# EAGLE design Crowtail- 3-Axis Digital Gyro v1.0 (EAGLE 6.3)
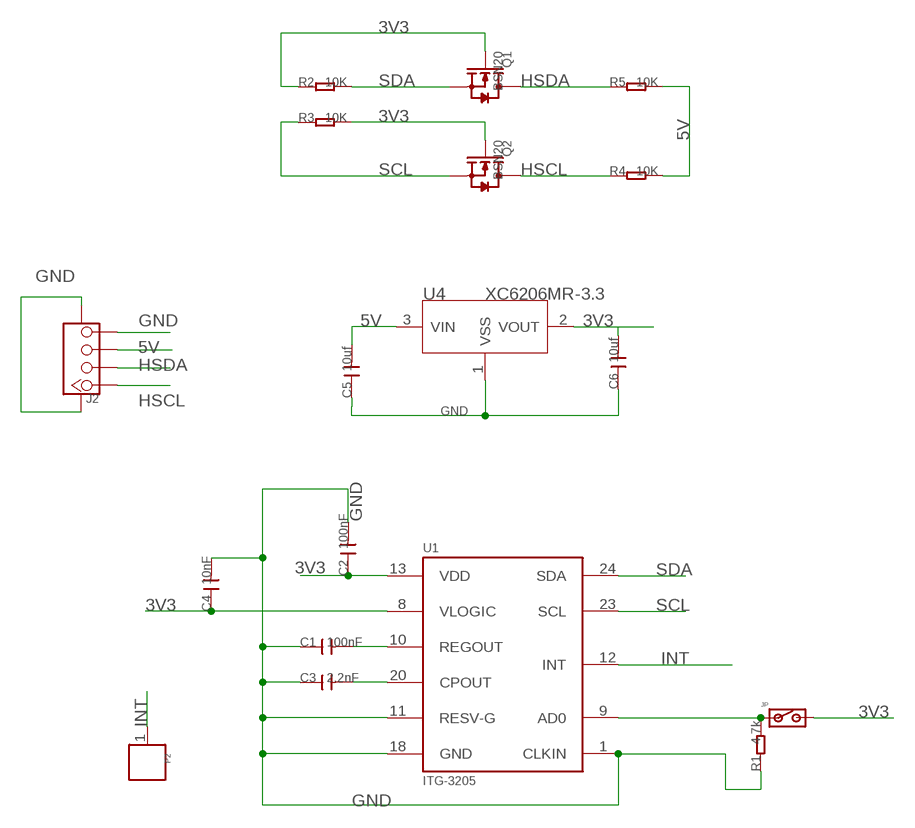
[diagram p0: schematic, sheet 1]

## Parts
C1  100nF  C-0603  [C0603]
C2  100nF  C-0603  [C0603]
C3  2.2nF  C-0603  [C0603]
C4  10nF  C-0603  [C0603]
C5  10uf  C-0603  [C0603]
C6  10uf  C-0603  [C0603]
J2  TWIG-4P-2.0-SMD-FEMALE-REINFORCE'DD'  [4P-SMD-2.0]
JP  DNP  JP_SW  [JP_SW]
P2  DNP  PAD'60/30'  [1P-65/35MIL]
Q1  BSN20  MOSFET-N'SOT23'  [SOT23]
Q2  BSN20  MOSFET-N'SOT23'  [SOT23]
R1  4.7k  R-0603  [R0603]
R2  10K  R-0603  [R0603]
R3  10K  R-0603  [R0603]
R4  10K  R-0603  [R0603]
R5  10K  R-0603  [R0603]
U1  ITG-3205  ITG-3200  [QFN-24]
U4  XC6206MR-3.3  XC6206MR  [SOT23]

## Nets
3V3: C2.1 C4.1 C6.2 JP.2 Q1.1(G) Q2.1(G) R2.1 R3.2 U1.8(VLOGIC) U1.13(VDD) U4.2(VOUT)
5V: C5.2 J2.3 R4.2 R5.2 U4.3(VIN)
GND: C1.1 C2.2 C3.1 C4.2 C5.1 C6.1 J2.4 J2.SS1 J2.SS2 R1.1 U1.1(CLKIN) U1.11(RESV-G) U1.18(GND) U4.1(VSS)
HSCL: J2.1 Q2.3(D) R4.1
HSDA: J2.2 Q1.3(D) R5.1
INT: P2.1 U1.12(INT)
N$2: C3.2 U1.20(CPOUT)
N$3: C1.2 U1.10(REGOUT)
N$4: JP.1 R1.2 U1.9(AD0)
SCL: Q2.2(S) R3.1 U1.23(SCL)
SDA: Q1.2(S) R2.2 U1.24(SDA)

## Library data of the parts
C1-C6 = Discrete:C*: Ceramic Capacitors
J2 = Connector:TWIG-4P-2.0-SMD-FEMALE-REINFORCE
JP = CPT_SMD:JP_SW
P2 = Discrete:PAD
Q1 Q2 = Discrete:MOSFET-N: IRLL014: http://www.vishay.com/docs/91319/sihll014.pdf
R1-R5 = Discrete:R*
U1 = IC:ITG-3200: ITG-3200 3-axis gyro, digital output, qfn24 package
U4 = IC:XC6206: LOW ESR Cap.Compatible Positive Voltage Regulators

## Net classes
0 default: width 0.203 mm, drill 0.305 mm, clearance 0.203 mm

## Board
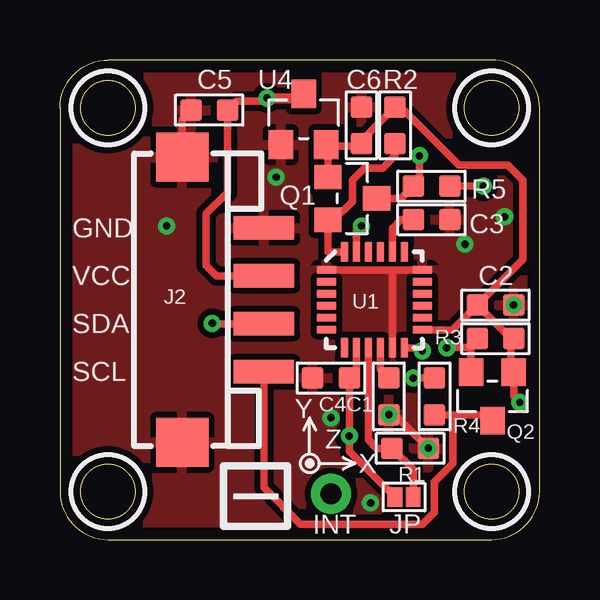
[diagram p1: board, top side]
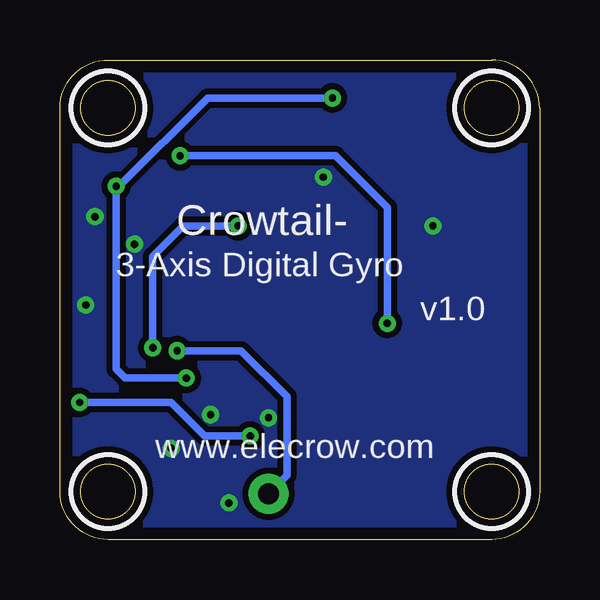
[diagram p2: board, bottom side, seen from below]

Size 20 x 20 mm. Coordinates in mm from the lower left corner, seen from the top.
Outline: 0,18 0,2 arc90 2,0 18,0 arc90 20,2 20,18 arc90 18,20 2,20 arc90 0,18
Outline: circle at 2,18 radius 1.14
Outline: circle at 2,2 radius 1.14
Outline: circle at 18,18 radius 1.14
Outline: circle at 18,2 radius 1.14
Copper layers (1*16): Top 0.035mm / dielectric 1.5mm / Bottom 0.035mm
Design rules "default *": minimum track width 10mil, minimum drill 12mil, track to track 8mil, track to pad 8mil, pad to pad 8mil, via to via 8mil, smd to smd 8mil, copper to edge 20mil, drill to drill 8mil, minimum pad ring 10mil, minimum via ring 8mil, stop-mask expansion 4mil, vias tented up to drill 100mil, thermal gap 10mil
tRestrict: area 0.5,16.5 to 3.5,19.5; area 0.5,0.5 to 3.5,3.5; area 16.5,16.5 to 19.5,19.5; area 16.5,0.5 to 19.5,3.5
bRestrict: area 0.5,16.5 to 3.5,19.5; area 0.5,0.5 to 3.5,3.5; area 16.5,16.5 to 19.5,19.5; area 16.5,0.5 to 19.5,3.5

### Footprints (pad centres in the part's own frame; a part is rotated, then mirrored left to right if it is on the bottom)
C0603 = smd 0.889 x 0.889: 1 -0.762,0; 2 0.762,0
4P-SMD-2.0 = smd 0.965 x 2.54: 1 -3,0; 2 -1,0; 3 1,0; 4 3,0 | smd 2.032 x 2.184: SS1 -5.946,3.4; SS2 5.946,3.4
JP_SW = smd 0.813 x 0.61: 1 0,0.381; 2 0,-0.381
1P-65/35MIL = drill 0.889 pad 1.651: 1 0,0
SOT23 = smd 1.016 x 1.143: 1 -0.889,-1.016; 2 0.889,-1.016; 3 0,1.016
R0603 = smd 0.889 x 0.889: 1 -0.762,0; 2 0.762,0
QFN-24 = smd 0.8 x 0.3: 1 -2,1.25; 2 -2,0.75; 3 -2,0.25; 4 -2,-0.25; 5 -2,-0.75; 6 -2,-1.25; 13 2,-1.25; 14 2,-0.75; 15 2,-0.25; 16 2,0.25; 17 2,0.75; 18 2,1.25 | smd 0.3 x 0.8: 7 -1.25,-2; 8 -0.75,-2; 9 -0.25,-2; 10 0.25,-2; 11 0.75,-2; 12 1.25,-2; 19 1.25,2; 20 0.75,2; 21 0.25,2; 22 -0.25,2; 23 -0.75,2; 24 -1.25,2
SOT23' = smd 1.016 x 1.2: 1 -0.95,-1.06; 2 0.95,-1.06; 3 0,1.06

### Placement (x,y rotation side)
C1  13.72,5.97 90 top
C2  18.16,9.78 0 top
C3  15.49,13.34 180 top
C4  11.3,6.73 180 top
C5  6.22,17.91 0 top
C6  12.57,17.27 270 top
J2  8.5,10 90 top
JP  14.35,1.78 270 top
P2  11.3,1.91 0 top
Q1  12.19,14.22 270 top
Q2  18.03,5.97 180 top
R1  14.61,3.81 180 top
R2  13.97,17.27 270 top
R3  18.16,8.38 0 top
R4  15.62,5.97 90 top
R5  15.49,14.73 0 top
U1  13.11,10 0 top
U4  XC6206MR-3.3  [SOT23']  10.16,17.53 0 top

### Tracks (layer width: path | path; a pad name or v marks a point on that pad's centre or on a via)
3V3  (via drill 0.3)
  Top 0.305: R3.2 18.8,8.38 | U1.13 16.37,8.75 C2.1 | Q1.1 11.18,16.4 | 11.18,16.4 U4.2 | C2.1 19.3,11.68 19.3,14.99 18.67,15.62 16.64,15.62 14.22,18.03 R2.1 12.57,16.64 C6.2 12.34,16.4 11.18,16.4 | U1.8 12.36,7.03 C4.1 v12.06,4.32 12.06,3.68 JP.2 | 18.8,8.38 18.8,7.11 Q2.1 18.92,5.97 v19.18,5.71 | 18.8,8.38 C2.1
  Bottom 0.305: v19.18,5.71 15.37,5.71 13.97,4.32 v12.06,4.32
5V  (via drill 0.3)
  Top 0.305: J2.3 6.53,11 6.1,11.43 6.1,13.59 6.99,14.48 C5.2 7.37,18.29 8.51,18.29 v8.64,18.41 9.99,18.41 U4.3 | R5.2 v17.65,14.73 | R4.2 v14.73,6.73
  Top 0.406: v8.64,18.41 10.16,18.41 U4.3
  Bottom 0.305: v8.64,18.41 13.84,18.41 17.53,14.73 v17.65,14.73 17.65,7.11 17.27,6.73 v14.73,6.73
GND  (via drill 0.3)
  Top 0.305: 11.86,11.25 U1.1 13.72,11.25 | 15.37,3.68 15.62,3.68 R1.1 13.97,5.21 C1.1 | J2.SS2 5.1,17.55 C5.1 | 13.72,11.25 U1.18 | U1.11 13.86,11.11 13.72,11.25
  other vias: 4.45,13.08 18.54,13.46 18.92,9.78 9.02,15.11 16.89,12.32 12.95,1.52 13.72,5.21 11.3,5.08 15.37,3.81
  pour Bottom (isolate 0.254): -0.51,-0.76 20.45,-0.89 20.32,20.32 -0.64,20.45
  pour Top (isolate 0.254): -0.51,-0.89 20.45,-0.89 20.32,20.45 -0.64,20.45
HSCL
  Top 0.305: R4.1 16.38,5.21 | 16.38,5.21 17.78,5.21 Q2.3 | J2.1 8.5,2.17 10.03,0.64 15.11,0.64 15.62,1.14 15.62,2.41 16.38,3.17 16.38,5.21
HSDA  (via drill 0.3)
  Top 0.305: Q1.3 14.22,14.22 R5.1 14.99,14.99 v14.99,16 | J2.2 6.35,9 v6.35,9.02
  Bottom 0.305: v6.35,9.02 6.35,13.84 8.51,16 v14.99,16
INT  (via drill 0.3)
  Top 0.305: U1.12 14.99,8 v15.11,7.87
  Bottom 0.305: v15.11,7.87 12.45,7.87 10.54,5.97 10.54,2.67 P2.1
N$2
  Top 0.305: U1.20 13.86,12.97 14.22,13.34 C3.2
N$3
  Top 0.305: U1.10 13.36,7.09 C1.2
N$4
  Top 0.305: U1.9 12.86,4.16 13.21,3.81 R1.2 14.73,2.92 JP.1
SCL  (via drill 0.3)
  Top 0.305: Q2.2 17.14,8.13 R3.1 17.02,8 v16.13,8 | U1.23 12.36,12.87 v12.57,13.08
  Bottom 0.305: v12.57,13.08 14.86,13.08 16.13,11.81 v16.13,8
SDA
  Top 0.305: U1.24 11.18,12 Q1.2 11.43,13.34 12.19,14.1 12.19,14.99 12.7,15.49 13.46,15.49 13.97,16 R2.2

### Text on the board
tPlace: GND | VCC | SDA | SCL | I
bPlace: Crowtail- | 3-Axis Digital Gyro | v1.0 | www.elecrow.com
tNames: Y | Z | X | INT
